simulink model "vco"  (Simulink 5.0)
settings: Solver=ode4  StartTime=0.0  StopTime=4  FixedStep=0.0002  RelTol=1e-6

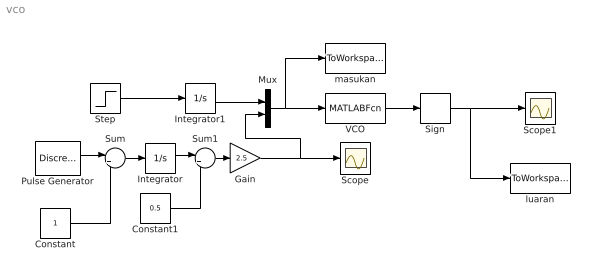
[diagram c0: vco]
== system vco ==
  Constant : Constant
  Constant1 : Constant  Value=0.5
  Gain : Gain  Gain=2.5
  Integrator : Integrator
  Integrator1 : Integrator
  Mux : Mux  Inputs=2
  Pulse Generator : DiscretePulseGenerator  PulseType=Time based  Amplitude=2  PulseWidth=50
  Scope : Scope
  Scope1 : Scope
  Sign : Signum
  Step : Step  Time=0  SampleTime=0
  Sum : Sum  Inputs=|+-
  Sum1 : Sum  Inputs=|+-
  VCO : MATLABFcn  MATLABFcn=vcomat
  luaran : ToWorkspace  VariableName=y  SampleTime=-1  SaveFormat=Array
  masukan : ToWorkspace  VariableName=x  SampleTime=-1  SaveFormat=Array
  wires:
  Pulse Generator/1 -> Sum/1
  Constant/1 -> Sum/2
  Sum/1 -> Integrator/1
  VCO/1 -> Sign/1
  Step/1 -> Integrator1/1
  Integrator1/1 -> Mux/1
  Mux/1 -> VCO/1, masukan/1
  Integrator/1 -> Sum1/1
  Constant1/1 -> Sum1/2
  Sum1/1 -> Gain/1
  Gain/1 -> Scope/1, Mux/2
  Sign/1 -> Scope1/1, luaran/1
